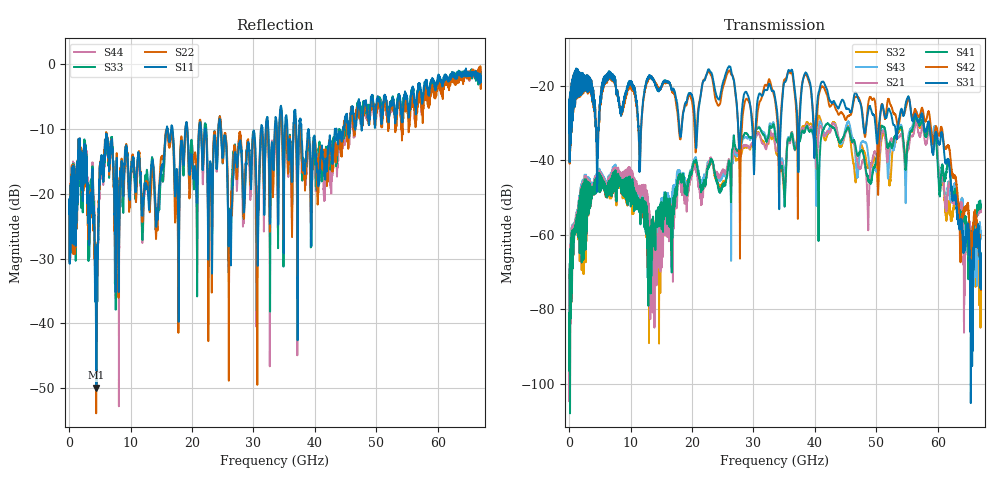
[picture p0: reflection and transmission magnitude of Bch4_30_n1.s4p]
!Agilent Technologies,N5247A,US51170199,A.09.90.13
!Agilent N5247A: A.09.90.13
!Date: Wednesday, October 17, 2018 17:53:10
!Correction: S11(Full 4 Port(1,2,3,4))
!S12(Full 4 Port(1,2,3,4))
!S13(Full 4 Port(1,2,3,4))
!S14(Full 4 Port(1,2,3,4))
!S21(Full 4 Port(1,2,3,4))
!S22(Full 4 Port(1,2,3,4))
!S23(Full 4 Port(1,2,3,4))
!S24(Full 4 Port(1,2,3,4))
!S31(Full 4 Port(1,2,3,4))
!S32(Full 4 Port(1,2,3,4))
!S33(Full 4 Port(1,2,3,4))
!S34(Full 4 Port(1,2,3,4))
!S41(Full 4 Port(1,2,3,4))
!S42(Full 4 Port(1,2,3,4))
!S43(Full 4 Port(1,2,3,4))
!S44(Full 4 Port(1,2,3,4))
!S4P File: Measurements: <S11,S12,S13,S14>,
!<S21,S22,S23,S24>,
!<S31,S32,S33,S34>,
!<S41,S42,S43,S44>:
# Hz S  dB  R 50
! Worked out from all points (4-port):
!   6701 points, 10 MHz to 67 GHz, reference 50 ohm
!   strongest paths, dB at 10 MHz, 16.76 GHz, 33.51 GHz, 50.25 GHz, 67 GHz:
!     S31: -32.6, -21.0, -23.0, -33.6, -74.6
!     S42: -32.7, -21.4, -23.8, -46.1, -75.0
!     S41: -81.0, -53.3, -32.9, -37.5, -52.1
!     S21: -75.9, -58.1, -35.4, -40.4, -53.4
!     S43: -85.3, -48.5, -31.7, -42.1, -59.5
!     S32: -93.2, -50.3, -35.7, -47.8, -78.9
!   lowest |S11| = -49.9 dB at 4.449 GHz (marker M1), VSWR 1.01, Z = 50 - j0.314 ohm
!   |S11| at or under -10 dB: start of sweep to 15.84 GHz; 24.7 GHz to 31.23 GHz (6.538 GHz wide, 23.4 % of centre); 38.95 GHz to 43.24 GHz (4.291 GHz wide, 10.4 % of centre)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
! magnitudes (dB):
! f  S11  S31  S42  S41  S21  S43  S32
! 10 MHz  -23.0  -32.6  -32.7  -81.0  -75.9  -85.3  -93.2
! 4.449 GHz  -49.9  -34.5  -33.3  -45.6  -45.1  -44.5  -45.6
! 6.039 GHz  -10.7  -17.2  -17.4  -47.0  -46.0  -45.6  -46.8
! 13.95 GHz  -20.3  -19.4  -19.2  -62.7  -62.3  -66.8  -66.2
! 30.65 GHz  -28.9  -24.1  -27.4  -31.5  -32.9  -31.3  -32.5
! 56.48 GHz  -6.0  -28.3  -27.1  -28.1  -29.6  -26.8  -27.7
! 67 GHz  -2.7  -74.6  -75.0  -52.1  -53.4  -59.5  -78.9
